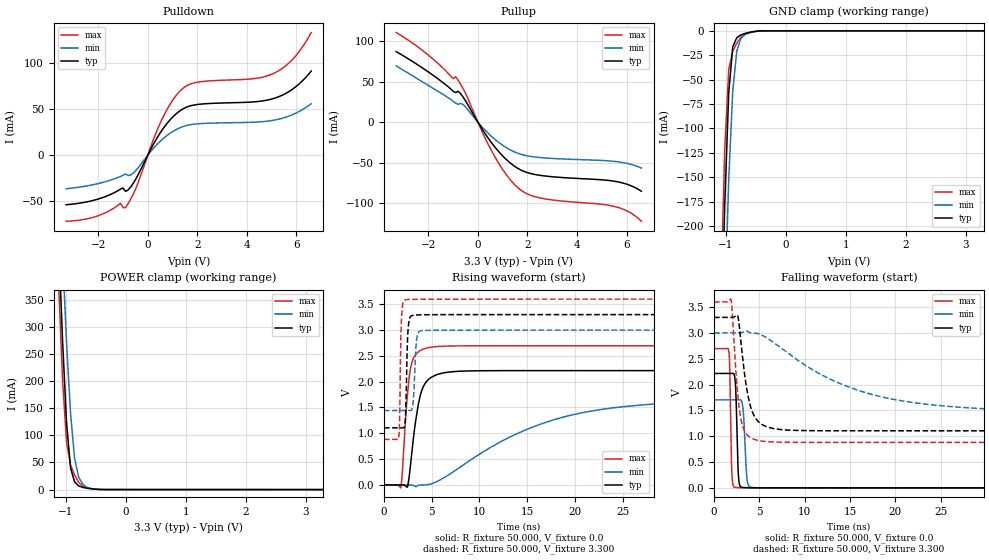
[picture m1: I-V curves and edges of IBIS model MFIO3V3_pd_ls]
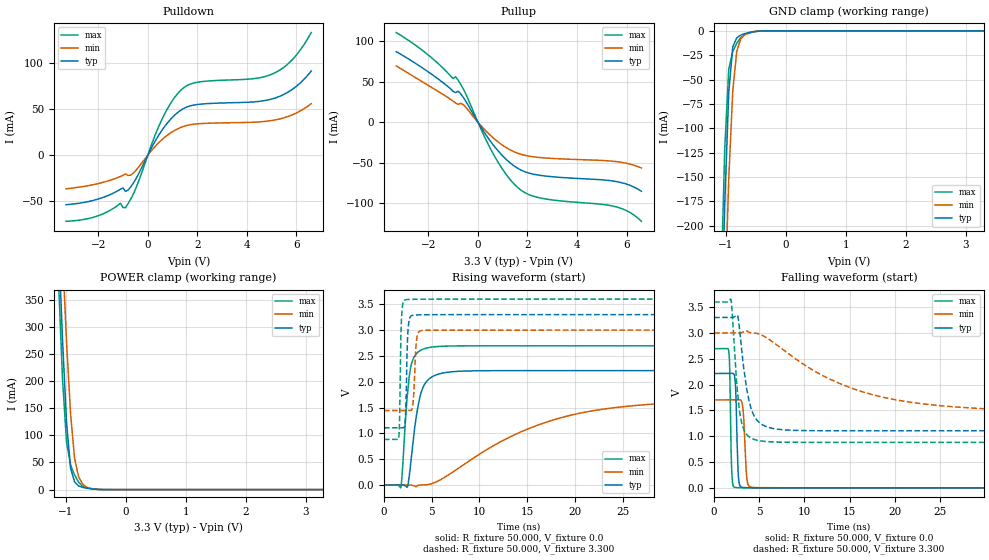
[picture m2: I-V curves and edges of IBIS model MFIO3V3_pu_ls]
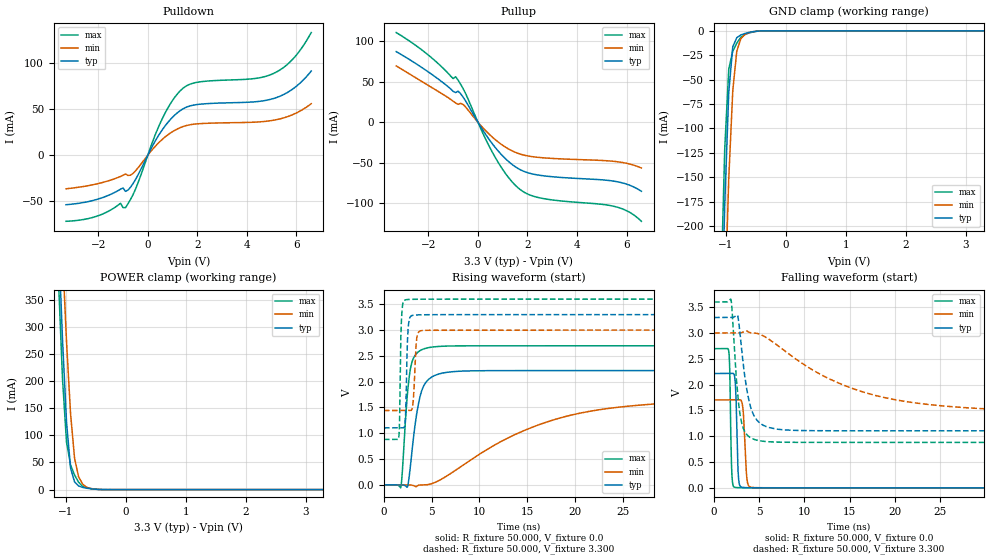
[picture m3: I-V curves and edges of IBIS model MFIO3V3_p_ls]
| IBIS file lpc551x_htqfp64.ibs
[IBIS Ver]   5.0
[File name]   lpc551x_htqfp64.ibs
[File Rev]   1.0
[Date]   June 22,2020
[Notes]   Rev History
|   1.0  initial release
[Disclaimer]   The model given below represents a 64-pin package.
[Copyright]   Copyright NXP 2020
[Component] lpc551x
[Manufacturer] NXP
[Package]
|   typ   min   max
R_pkg   0.19702   0.096175   0.23367
L_pkg   3.574e-9   2.964e-9   4.311e-9
C_pkg   4.829e-13   4.303e-13   6.109e-13
[Pin]   signal_name   model_name   R_pin   L_pin   C_pin
9   VDDA   POWER   NA   NA   NA
25   VBUS   POWER   0.20915   3.347e-9   4.679e-13
27   USB1_3V3   POWER   NA   NA   NA
61   USB0_3V3   POWER   NA   NA   NA
8   VDDE   POWER   NA   NA   NA
16   VDDE   POWER   NA   NA   NA
43   VDDE   POWER   NA   NA   NA
54   VDDE   POWER   NA   NA   NA
28   VDD_PMU   POWER   NA   NA   NA
10   VREFP   POWER   0.18173   2.964e-9   4.54e-13
32   VBAT_DCDC_CORE   POWER   0.096175   3.194e-9   6.109e-13
33   VBAT_PMU   POWER   0.21402   4.013e-9   4.752e-13
24   USB1_DM   NC   0.20325   3.453e-9   4.718e-13
23   USB1_DP   NC   0.21049   3.339e-9   4.746e-13
29   FB   NC   NA   NA   NA
31   LX   NC   0.12749   3.011e-9   5.849e-13
36   P0_0   gpio3v3   0.18524   3.505e-9 4.679e-13
2   P0_1   gpio3v3   0.21276   3.977e-9 5.283e-13
52   P0_2   gpio3v3   0.20828   3.749e-9 4.838e-13
53   P0_3   gpio3v3   0.20955   3.477e-9 4.766e-13
55   P0_4   gpio3v3   0.20447   3.499e-9 4.566e-13
56   P0_5   gpio3v3   0.20052   3.543e-9  4.69e-13
57   P0_6   gpio3v3   0.20007   3.565e-9 4.736e-13
1   P0_7   gpio3v3   0.22847   4.288e-9 5.092e-13
17   P0_8   gpio3v3   0.22136   4.132e-9 4.883e-13
37   P0_9   gpio3v3   0.1773   3.36e-9 4.575e-13
13   P0_10   gpio3v3   0.18906   3.545e-9 4.881e-13
6   P0_11   gpio3v3   0.17925   3.357e-9  4.61e-13
5   P0_12   gpio3v3   0.18582   3.52e-9  4.76e-13
46   P0_13   iicgpio3v3   0.19221   3.582e-9 4.844e-13
47   P0_14   iicgpio3v3   0.20296   3.765e-9 4.948e-13
14   P0_15   gpio3v3   0.19983   3.666e-9 5.083e-13
7   P0_16   gpio3v3   0.17909   3.101e-9 4.519e-13
3   P0_17   gpio3v3   0.20017   3.778e-9 4.971e-13
38   P0_18   gpio3v3   0.17183   3.265e-9 4.388e-13
58   P0_19   gpio3v3   0.20259   3.636e-9 4.686e-13
48   P0_20   gpio3v3   0.21365   4.055e-9 4.764e-13
49   P0_21   gpio3v3   0.22994   4.311e-9 4.976e-13
50   P0_22   gpio3v3   0.2203   4.016e-9 5.173e-13
12   P0_23   gpio3v3   0.1835   3.254e-9 4.662e-13
45   P0_24   gpio3v3   0.18339   3.43e-9 4.615e-13
51   P0_25   gpio3v3   0.21235   3.87e-9 5.028e-13
40   P0_26   gpio3v3   0.16841   3.135e-9 4.403e-13
18   P0_27   gpio3v3   0.21181   3.898e-9 4.964e-13
44   P0_28   gpio3v3   0.18479   3.216e-9 4.418e-13
59   P0_29   gpio3v3   0.20617   3.657e-9  4.73e-13
60   P0_30   gpio3v3   0.21575   3.597e-9 4.783e-13
15   P0_31   gpio3v3   0.21765   3.65e-9 5.199e-13
4   P1_0   gpio3v3   0.19509   3.68e-9 4.803e-13
39   P1_1   gpio3v3   0.16986   3.202e-9 4.303e-13
41   P1_2   gpio3v3   0.17055   3.135e-9 4.429e-13
42   P1_3   gpio3v3   0.17903   3.13e-9 4.331e-13
21   RESETN   gpio3v3   0.21486   3.524e-9 4.684e-13
63   USB0_DM   NC   0.23367   3.701e-9   5.248e-13
62   USB0_DP   NC   0.23063   3.603e-9   5.115e-13
35   XTAL32K_N   NC   0.19233   3.61e-9   4.888e-13
34   XTAL32K_P   NC   0.20386   3.799e-9   5.036e-13
19   XTAL32M_N   NC   0.21308   3.871e-9   4.912e-13
20   XTAL32M_P   NC   0.2074   3.75e-9   4.799e-13
65   VSS   GND   NA   NA   NA
11   VSSA   GND   NA   NA   NA
22   USB1_VSS   GND   NA   NA   NA
26   USB1_VSS   GND   NA   NA   NA
30   VSS_DCDC   GND   NA   NA   NA
64   USB0_VSS   GND   NA   NA   NA
|   Model Selector
[Model Selector] gpio3v3
MFIO3V3_pd_hs  EPUN=1 EPD=1 EHS=1
MFIO3V3_pd_ls  EPUN=1 EPD=1 EHS=0
MFIO3V3_pu_hs  EPUN=0 EPD=0 EHS=1
MFIO3V3_pu_ls  EPUN=0 EPD=0 EHS=0
MFIO3V3_p_hs  EPUN=1 EPD=0 EHS=1
MFIO3V3_p_ls  EPUN=1 EPD=0 EHS=0
MFIO3V3_r_hs  EPUN=0 EPD=1 EHS=1
MFIO3V3_r_ls  EPUN=0 EPD=1 EHS=0
[Model Selector] iicgpio3v3
IIC3V3_pd_hs  EGP=1 EPUN=1 EPD=1 EHS=1
IIC3V3_pd_ls  EGP=1 EPUN=1 EPD=1 EHS=0
IIC3V3_p_hs  EGP=1 EPUN=1 EPD=0 EHS=1
IIC3V3_p_ls  EGP=1 EPUN=1 EPD=0 EHS=0
IIC3V3_pu_hs  EGP=1 EPUN=0 EPD=0 EHS=1
IIC3V3_pu_ls  EGP=1 EPUN=0 EPD=0 EHS=0
IIC3V3_r_hs  EGP=1 EPUN=0 EPD=1 EHS=1
IIC3V3_r_ls  EGP=1 EPUN=0 EPD=1 EHS=0
IIC3V3_pd_iic_hs  EGP=0 ECS=0 EPUN=1 EPD=1
IIC3V3_p_iic_hs  EGP=0 ECS=0 EPUN=1 EPD=0
IIC3V3_pu_iic_hs  EGP=0 ECS=0 EPUN=0 EPD=0
IIC3V3_r_iic_hs  EGP=0 ECS=0 EPUN=0 EPD=1
IIC3V3_pd_iic_pu_hs  EGP=0 ECS=1 EPUN=1 EPD=1  SSEL=1
IIC3V3_p_iic_pu_hs  EGP=0 ECS=1 EPUN=1 EPD=0  SSEL=1
IIC3V3_pu_iic_pu_hs  EGP=0 ECS=1 EPUN=0 EPD=0  SSEL=1
IIC3V3_r_iic_pu_hs  EGP=0 ECS=1 EPUN=0 EPD=1  SSEL=1
| Models and submodels in the file (24): MFIO3V3_pd_hs (I/O), MFIO3V3_pd_ls (I/O), MFIO3V3_pu_hs (I/O), MFIO3V3_pu_ls (I/O), MFIO3V3_p_hs (I/O), MFIO3V3_p_ls (I/O), MFIO3V3_r_hs (I/O), MFIO3V3_r_ls (I/O), IIC3V3_pd_hs (I/O), IIC3V3_pd_ls (I/O), IIC3V3_p_hs (I/O), IIC3V3_p_ls (I/O), IIC3V3_pu_hs (I/O), IIC3V3_pu_ls (I/O), IIC3V3_r_hs (I/O), IIC3V3_r_ls (I/O), IIC3V3_pd_iic_hs (I/O_open_drain), IIC3V3_p_iic_hs (I/O_open_drain), IIC3V3_pu_iic_hs (I/O_open_drain), IIC3V3_r_iic_hs (I/O_open_drain), IIC3V3_pd_iic_pu_hs (I/O_open_drain), IIC3V3_p_iic_pu_hs (I/O_open_drain), IIC3V3_pu_iic_pu_hs (I/O_open_drain), IIC3V3_r_iic_pu_hs (I/O_open_drain)
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|   Model MFIO3V3_pd_ls
[Model] MFIO3V3_pd_ls
Model_type I/O
Polarity   Non-Inverting
Enable   Active-Low
Vinl =  0.990V
Vinh =  2.310V
Vmeas =  1.650V
Cref =  0.0F
Rref =  100.000
Vref =  0.0V
C_comp   1.906pF   1.877pF   1.925pF
C_comp_pullup   1.141pF   1.113pF   1.145pF
C_comp_pulldown   0.641pF   0.601pF   0.647pF
[Model Spec]
Vinh   2.310V   2.100V   2.520V
Vinl   0.990V   0.900V   1.080V
Vmeas   1.650V   1.500V   1.800V
Vref   0.0V   0.0V   0.0V
Cref   0.0F   0.0F   0.0F
Rref   100.000   100.000   100.000
[Temperature Range]   25.000   0.125k   -40.000
[Voltage Range]   3.300V   3.000V   3.600V
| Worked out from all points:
|   slope of the pulldown table from 0 to 0.495 V, typ, clamps not added: 20.7 ohm
|   slope of the pullup table from 0 to 0.495 V, typ, clamps not added: 21.4 ohm
|   GND clamp passes 1 mA (typ) near -0.56 V on its own axis
|   POWER clamp passes 1 mA (typ) near -0.53 V on its own axis
|   rising waveform, R_fixture 50.000, V_fixture 0.0: 20-80 % time 1.05ns typ, 11.9ns min, 670ps max; typ from 0 V to 2.21 V
|   rising waveform, R_fixture 50.000, V_fixture 3.300: 20-80 % time 176ps typ, 234ps min, 146ps max; typ from 1.1 V to 3.3 V
|   falling waveform, R_fixture 50.000, V_fixture 0.0: 20-80 % time 203ps typ, 279ps min, 162ps max; typ from 2.21 V to 0 V
|   falling waveform, R_fixture 50.000, V_fixture 3.300: 20-80 % time 1.13ns typ, 11.2ns min, 744ps max; typ from 3.3 V to 1.1 V
[Pulldown]
|Voltage   I(typ)   I(min)   I(max)
-3.3V     -53.7mA    -36.43mA   -71.67mA
-2.1V     -48.29mA   -31.37mA   -66.51mA
-1.1V     -36.82mA   -23.05mA   -52.1mA
-900mV    -39.2mA    -20.39mA   -56.91mA
-600mV    -30.96mA   -19.83mA   -42.97mA
600mV     28.07mA    17.5mA     40.4mA
1V        41.17mA    25.53mA    59.41mA
1.4V      49.87mA    30.79mA    72.04mA
2V        54.93mA    33.94mA    79.03mA
5V        60.84mA    37.53mA    87.68mA
5.9V      72.62mA    44.52mA    105.4mA
6.6V      91.19mA    55.78mA    132.9mA
[Pullup]
|Voltage   I(typ)   I(min)   I(max)
-3.3V     87.16mA    69.54mA    110.7mA
-2.1V     64.12mA    47.22mA    85.31mA
-1V       38.1mA     25.85mA    53.88mA
-900mV    36.64mA    23.75mA    56.16mA
-800mV    38.25mA    22.02mA    51.93mA
-600mV    31.06mA    21.93mA    41.58mA
700mV     -31.25mA   -21.55mA   -43.56mA
1.2V      -47.6mA    -32.42mA   -66.97mA
1.7V      -58.52mA   -39.3mA    -83.05mA
2.6V      -66.01mA   -43.88mA   -94.06mA
5.6V      -73.4mA    -48.74mA   -104.7mA
6.6V      -85.32mA   -56.6mA    -122.4mA
[GND_clamp]
|Voltage   I(typ)   I(min)   I(max)
-3.3V     -7.222A    -7.177A    -7.278A
-1.089V   -337.1mA   -440.8mA   -274.1mA
-1.022V   -178.2mA   -284.2mA   -121mA
-955mV    -63.05mA   -151.6mA   -39.25mA
-888mV    -16.33mA   -61.34mA   -20.9mA
-821mV    -7.066mA   -20.84mA   -12.66mA
-754mV    -4.265mA   -8.157mA   -6.693mA
-687mV    -2.794mA   -3.896mA   -3.841mA
-620mV    -1.725mA   -1.894mA   -2.339mA
-419mV    -112.4uA   -138.2uA   -135uA
3.3V      0A         0A         0A
[POWER_clamp]
|Voltage   I(typ)   I(min)   I(max)
-3.3V     8.016A     7.986A     8.074A
-1.122V   463.8mA    614.4mA    385mA
-1.055V   276.3mA    435mA      203.9mA
-988mV    124.1mA    272.4mA    87.22mA
-921mV    40.03mA    140.2mA    45.68mA
-854mV    14.24mA    57.83mA    27.12mA
-787mV    6.921mA    23.8mA     13.77mA
-720mV    4.141mA    10.27mA    6.207mA
-653mV    2.682mA    4.42mA     3.699mA
-586mV    1.616mA    1.919mA    2.191mA
-452mV    346.9uA    411.9uA    422.9uA
3.3V      0A         0A         0A
[Ramp]
| variable   typ   min   max
dV/dt_r   1.328/1.048n   1.021/11.887n   1.617/0.670n
dV/dt_f   1.317/1.132n   0.935/11.171n   1.631/0.743n
R_load = 50.000
[Rising Waveform]
R_fixture= 50.000
V_fixture= 0.0
V_fixture_min= 0.0
V_fixture_max= 0.0
|time   V(typ)   V(min)   V(max)
0s        11.38nV    124.8nV    46.5nV
1.76ns    11.77uV    -379.4nV   -52.39mV
1.89ns    124.5uV    -254.1nV   156mV
2.47ns    -34.09mV   65.71uV    1.767V
2.93ns    642.6mV    -4.824mV   2.378V
3.75ns    1.693V     -3.224mV   2.598V
4.9ns     2.078V     17.79mV    2.667V
15.38ns   2.214V     1.106V     2.695V
25.84ns   2.214V     1.529V     2.695V
100ns     2.214V     1.702V     2.695V
[Rising Waveform]
R_fixture= 50.000
V_fixture= 3.300
V_fixture_min= 3.000
V_fixture_max= 3.600
|time   V(typ)   V(min)   V(max)
0s        1.105V     1.44V      880.4mV
1.55ns    1.105V     1.44V      919.2mV
1.85ns    1.105V     1.44V      3.271V
2.2ns     1.184V     1.44V      3.582V
2.34ns    1.855V     1.44V      3.589V
2.64ns    3.192V     1.44V      3.594V
3.07ns    3.287V     1.621V     3.596V
3.43ns    3.293V     2.839V     3.597V
4.06ns    3.296V     2.992V     3.598V
100ns     3.299V     2.999V     3.599V
[Falling Waveform]
R_fixture= 50.000
V_fixture= 0.0
V_fixture_min= 0.0
V_fixture_max= 0.0
|time   V(typ)   V(min)   V(max)
0s        2.214V     1.703V     2.695V
1.63ns    2.214V     1.703V     2.64V
1.73ns    2.214V     1.703V     2.3V
1.97ns    2.214V     1.703V     263mV
2.38ns    1.941V     1.702V     7.184mV
2.7ns     199.7mV    1.703V     3.012mV
3.2ns     7.193mV    1.527V     1.541mV
3.63ns    2.938mV    178.8mV    1.008mV
4.26ns    1.462mV    6.421mV    552.8uV
100ns     15.88nV    209.7nV    49.27nV
[Falling Waveform]
R_fixture= 50.000
V_fixture= 3.300
V_fixture_min= 3.000
V_fixture_max= 3.600
|time   V(typ)   V(min)   V(max)
0s        3.299V     2.999V     3.599V
1.87ns    3.299V     2.999V     3.646V
2.6ns     3.336V     2.999V     1.836V
3.1ns     2.603V     3.009V     1.222V
3.85ns    1.693V     3.011V     992.4mV
4.41ns    1.398V     2.998V     939.4mV
5.16ns    1.242V     2.965V     908.2mV
14.39ns   1.105V     1.984V     880.4mV
25.09ns   1.105V     1.589V     880.4mV
100ns     1.105V     1.44V      880.4mV
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|   Model MFIO3V3_pu_ls
[Model] MFIO3V3_pu_ls
Model_type I/O
Polarity   Non-Inverting
Enable   Active-Low
Vinl =  0.990V
Vinh =  2.310V
Vmeas =  1.650V
Cref =  0.0F
Rref =  100.000
Vref =  0.0V
C_comp   1.906pF   1.877pF   1.925pF
C_comp_pullup   1.139pF   1.112pF   1.144pF
C_comp_pulldown   0.643pF   0.602pF   0.649pF
[Model Spec]
Vinh   2.310V   2.100V   2.520V
Vinl   0.990V   0.900V   1.080V
Vmeas   1.650V   1.500V   1.800V
Vref   0.0V   0.0V   0.0V
Cref   0.0F   0.0F   0.0F
Rref   100.000   100.000   100.000
[Temperature Range]   25.000   0.125k   -40.000
[Voltage Range]   3.300V   3.000V   3.600V
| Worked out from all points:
|   slope of the pulldown table from 0 to 0.495 V, typ, clamps not added: 20.7 ohm
|   slope of the pullup table from 0 to 0.495 V, typ, clamps not added: 21.4 ohm
|   GND clamp passes 1 mA (typ) near -0.55 V on its own axis
|   POWER clamp passes 1 mA (typ) near -0.54 V on its own axis
|   rising waveform, R_fixture 50.000, V_fixture 0.0: 20-80 % time 1.05ns typ, 11.9ns min, 674ps max; typ from 0.001 V to 2.21 V
|   rising waveform, R_fixture 50.000, V_fixture 3.300: 20-80 % time 179ps typ, 230ps min, 146ps max; typ from 1.11 V to 3.3 V
|   falling waveform, R_fixture 50.000, V_fixture 0.0: 20-80 % time 203ps typ, 278ps min, 162ps max; typ from 2.21 V to 0.001 V
|   falling waveform, R_fixture 50.000, V_fixture 3.300: 20-80 % time 1.14ns typ, 11.2ns min, 744ps max; typ from 3.3 V to 1.11 V
[Pulldown]
|Voltage   I(typ)   I(min)   I(max)
-3.3V     -53.7mA    -36.43mA   -71.67mA
-2.1V     -48.29mA   -31.37mA   -66.51mA
-1.1V     -36.82mA   -23.05mA   -52.1mA
-900mV    -39.2mA    -20.39mA   -56.91mA
-600mV    -30.96mA   -19.83mA   -42.97mA
600mV     28.07mA    17.5mA     40.4mA
1V        41.17mA    25.53mA    59.41mA
1.4V      49.87mA    30.79mA    72.04mA
2V        54.93mA    33.94mA    79.03mA
5V        60.84mA    37.53mA    87.68mA
5.9V      72.62mA    44.52mA    105.4mA
6.6V      91.19mA    55.78mA    132.9mA
[Pullup]
|Voltage   I(typ)   I(min)   I(max)
-3.3V     87.16mA    69.54mA    110.7mA
-2.1V     64.12mA    47.22mA    85.31mA
-1V       38.1mA     25.85mA    53.88mA
-900mV    36.64mA    23.75mA    56.16mA
-800mV    38.25mA    22.02mA    51.93mA
-600mV    31.06mA    21.93mA    41.58mA
700mV     -31.25mA   -21.55mA   -43.56mA
1.2V      -47.6mA    -32.42mA   -66.97mA
1.7V      -58.52mA   -39.3mA    -83.05mA
2.6V      -66.01mA   -43.88mA   -94.06mA
5.6V      -73.4mA    -48.74mA   -104.7mA
6.6V      -85.32mA   -56.6mA    -122.4mA
[GND_clamp]
|Voltage   I(typ)   I(min)   I(max)
-3.3V     -7.222A    -7.177A    -7.278A
-1.089V   -337.2mA   -440.9mA   -274.2mA
-1.022V   -178.3mA   -284.2mA   -121.1mA
-955mV    -63.12mA   -151.7mA   -39.33mA
-888mV    -16.39mA   -61.39mA   -20.98mA
-821mV    -7.132mA   -20.89mA   -12.74mA
-754mV    -4.331mA   -8.209mA   -6.777mA
-687mV    -2.86mA    -3.948mA   -3.925mA
-620mV    -1.791mA   -1.946mA   -2.423mA
-419mV    -178.1uA   -190.3uA   -219.1uA
3.3V      0A         0A         0A
[POWER_clamp]
|Voltage   I(typ)   I(min)   I(max)
-3.3V     8.016A     7.986A     8.074A
-1.122V   463.7mA    614.3mA    385mA
-1.055V   276.3mA    434.9mA    203.9mA
-988mV    124mA      272.3mA    87.13mA
-921mV    39.96mA    140.1mA    45.6mA
-854mV    14.17mA    57.77mA    27.03mA
-787mV    6.855mA    23.75mA    13.68mA
-720mV    4.075mA    10.22mA    6.123mA
-653mV    2.616mA    4.368mA    3.615mA
-586mV    1.55mA     1.867mA    2.107mA
-452mV    281.1uA    359.9uA    338.7uA
3.3V      0A         0A         0A
[Ramp]
| variable   typ   min   max
dV/dt_r   1.329/1.048n   1.022/11.881n   1.617/0.670n
dV/dt_f   1.316/1.133n   0.935/11.179n   1.631/0.744n
R_load = 50.000
[Rising Waveform]
R_fixture= 50.000
V_fixture= 0.0
V_fixture_min= 0.0
V_fixture_max= 0.0
|time   V(typ)   V(min)   V(max)
0s        869.8uV    949.2uV    842.8uV
1.76ns    883.1uV    948.8uV    -50.04mV
1.91ns    1.009mV    949.1uV    208mV
2.46ns    -36.02mV   1.012mV    1.752V
2.89ns    574.4mV    -2.122mV   2.352V
3.71ns    1.664V     -1.354mV   2.595V
4.93ns    2.083V     22.11mV    2.669V
15.41ns   2.215V     1.111V     2.696V
25.89ns   2.215V     1.532V     2.696V
100ns     2.215V     1.704V     2.696V
[Rising Waveform]
R_fixture= 50.000
V_fixture= 3.300
V_fixture_min= 3.000
V_fixture_max= 3.600
|time   V(typ)   V(min)   V(max)
0s        1.106V     1.442V     881.7mV
1.55ns    1.106V     1.442V     920.7mV
1.83ns    1.106V     1.442V     3.201V
2.2ns     1.19V      1.442V     3.584V
2.36ns    2.014V     1.442V     3.591V
2.67ns    3.219V     1.441V     3.595V
3.05ns    3.288V     1.591V     3.597V
3.47ns    3.295V     2.885V     3.598V
4.05ns    3.297V     2.994V     3.599V
100ns     3.3V       3V         3.6V
[Falling Waveform]
R_fixture= 50.000
V_fixture= 0.0
V_fixture_min= 0.0
V_fixture_max= 0.0
|time   V(typ)   V(min)   V(max)
0s        2.215V     1.704V     2.696V
1.63ns    2.215V     1.704V     2.641V
1.73ns    2.215V     1.704V     2.3V
1.97ns    2.216V     1.704V     265.9mV
2.37ns    1.988V     1.704V     8.752mV
2.68ns    252.6mV    1.704V     4.211mV
3.22ns    8.138mV    1.493V     2.448mV
3.64ns    3.966mV    165.1mV    1.883mV
4.28ns    2.4mV      8.68mV     1.408mV
100ns     869.8uV    949.4uV    842.8uV
[Falling Waveform]
R_fixture= 50.000
V_fixture= 3.300
V_fixture_min= 3.000
V_fixture_max= 3.600
|time   V(typ)   V(min)   V(max)
0s        3.3V       3V         3.6V
1.88ns    3.3V       3V         3.639V
2.61ns    3.334V     3V         1.817V
3.06ns    2.664V     3.008V     1.251V
3.83ns    1.711V     3.015V     996.5mV
4.37ns    1.414V     3.001V     943.5mV
5.06ns    1.258V     2.975V     912.3mV
14.38ns   1.106V     1.987V     881.7mV
25.08ns   1.106V     1.591V     881.7mV
100ns     1.106V     1.442V     881.7mV
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|   Model MFIO3V3_p_ls
[Model] MFIO3V3_p_ls
Model_type I/O
Polarity   Non-Inverting
Enable   Active-Low
Vinl =  0.990V
Vinh =  2.310V
Vmeas =  1.650V
Cref =  0.0F
Rref =  100.000
Vref =  0.0V
C_comp   1.906pF   1.877pF   1.925pF
C_comp_pullup   1.140pF   1.112pF   1.144pF
C_comp_pulldown   0.642pF   0.602pF   0.649pF
[Model Spec]
Vinh   2.310V   2.100V   2.520V
Vinl   0.990V   0.900V   1.080V
Vmeas   1.650V   1.500V   1.800V
Vref   0.0V   0.0V   0.0V
Cref   0.0F   0.0F   0.0F
Rref   100.000   100.000   100.000
[Temperature Range]   25.000   0.125k   -40.000
[Voltage Range]   3.300V   3.000V   3.600V
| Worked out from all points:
|   slope of the pulldown table from 0 to 0.495 V, typ, clamps not added: 20.7 ohm
|   slope of the pullup table from 0 to 0.495 V, typ, clamps not added: 21.4 ohm
|   GND clamp passes 1 mA (typ) near -0.56 V on its own axis
|   POWER clamp passes 1 mA (typ) near -0.54 V on its own axis
|   rising waveform, R_fixture 50.000, V_fixture 0.0: 20-80 % time 1.05ns typ, 11.9ns min, 670ps max; typ from 0 V to 2.21 V
|   rising waveform, R_fixture 50.000, V_fixture 3.300: 20-80 % time 177ps typ, 237ps min, 147ps max; typ from 1.1 V to 3.3 V
|   falling waveform, R_fixture 50.000, V_fixture 0.0: 20-80 % time 203ps typ, 282ps min, 162ps max; typ from 2.21 V to 0 V
|   falling waveform, R_fixture 50.000, V_fixture 3.300: 20-80 % time 1.14ns typ, 11.2ns min, 740ps max; typ from 3.3 V to 1.1 V
[Pulldown]
|Voltage   I(typ)   I(min)   I(max)
-3.3V     -53.7mA    -36.43mA   -71.67mA
-2.1V     -48.29mA   -31.37mA   -66.51mA
-1.1V     -36.82mA   -23.05mA   -52.1mA
-900mV    -39.2mA    -20.39mA   -56.91mA
-600mV    -30.96mA   -19.83mA   -42.97mA
600mV     28.07mA    17.5mA     40.4mA
1V        41.17mA    25.53mA    59.41mA
1.4V      49.87mA    30.79mA    72.04mA
2V        54.93mA    33.94mA    79.03mA
5V        60.84mA    37.53mA    87.68mA
5.9V      72.62mA    44.52mA    105.4mA
6.6V      91.19mA    55.78mA    132.9mA
[Pullup]
|Voltage   I(typ)   I(min)   I(max)
-3.3V     87.16mA    69.54mA    110.7mA
-2.1V     64.12mA    47.22mA    85.31mA
-1V       38.1mA     25.85mA    53.88mA
-900mV    36.64mA    23.75mA    56.16mA
-800mV    38.25mA    22.02mA    51.93mA
-600mV    31.06mA    21.93mA    41.58mA
700mV     -31.25mA   -21.55mA   -43.56mA
1.2V      -47.6mA    -32.42mA   -66.97mA
1.7V      -58.52mA   -39.3mA    -83.05mA
2.6V      -66.01mA   -43.88mA   -94.06mA
5.6V      -73.4mA    -48.74mA   -104.7mA
6.6V      -85.32mA   -56.6mA    -122.4mA
[GND_clamp]
|Voltage   I(typ)   I(min)   I(max)
-3.3V     -7.222A    -7.177A    -7.278A
-1.089V   -337.1mA   -440.8mA   -274.1mA
-1.022V   -178.2mA   -284.2mA   -121mA
-955mV    -63.04mA   -151.6mA   -39.24mA
-888mV    -16.32mA   -61.33mA   -20.89mA
-821mV    -7.057mA   -20.83mA   -12.64mA
-754mV    -4.256mA   -8.15mA    -6.682mA
-687mV    -2.785mA   -3.888mA   -3.83mA
-620mV    -1.717mA   -1.887mA   -2.329mA
-419mV    -104.8uA   -131.8uA   -126uA
3.3V      0A         0A         0A
[POWER_clamp]
|Voltage   I(typ)   I(min)   I(max)
-3.3V     8.016A     7.986A     8.074A
-1.122V   463.7mA    614.3mA    384.9mA
-1.055V   276.2mA    434.9mA    203.8mA
-988mV    124mA      272.3mA    87.12mA
-921mV    39.95mA    140.1mA    45.59mA
-854mV    14.16mA    57.77mA    27.02mA
-787mV    6.846mA    23.74mA    13.67mA
-720mV    4.066mA    10.21mA    6.113mA
-653mV    2.607mA    4.361mA    3.605mA
-586mV    1.542mA    1.86mA     2.097mA
-452mV    273.4uA    353.7uA    329.6uA
3.3V      0A         0A         0A
[Ramp]
| variable   typ   min   max
dV/dt_r   1.329/1.049n   1.022/11.884n   1.618/0.670n
dV/dt_f   1.317/1.134n   0.935/11.178n   1.632/0.744n
R_load = 50.000
[Rising Waveform]
R_fixture= 50.000
V_fixture= 0.0
V_fixture_min= 0.0
V_fixture_max= 0.0
|time   V(typ)   V(min)   V(max)
0s        11.91nV    127.2nV    48.18nV
1.76ns    14.07uV    -353.2nV   -52.48mV
1.9ns     130.3uV    -106.1nV   185.6mV
2.46ns    -38.99mV   62.57uV    1.761V
2.93ns    644.9mV    -4.797mV   2.378V
3.65ns    1.606V     -5.408mV   2.586V
4.94ns    2.084V     20.24mV    2.669V
15.63ns   2.215V     1.125V     2.696V
25.83ns   2.215V     1.53V      2.696V
100ns     2.215V     1.703V     2.696V
[Rising Waveform]
R_fixture= 50.000
V_fixture= 3.300
V_fixture_min= 3.000
V_fixture_max= 3.600
|time   V(typ)   V(min)   V(max)
0s        1.105V     1.441V     880.7mV
1.55ns    1.105V     1.441V     919.6mV
1.84ns    1.105V     1.441V     3.233V
2.22ns    1.224V     1.441V     3.584V
2.37ns    2.139V     1.441V     3.59V
2.68ns    3.224V     1.44V      3.594V
3.06ns    3.287V     1.603V     3.596V
3.45ns    3.294V     2.861V     3.598V
4.07ns    3.297V     2.993V     3.599V
100ns     3.3V       3V         3.6V
[Falling Waveform]
R_fixture= 50.000
V_fixture= 0.0
V_fixture_min= 0.0
V_fixture_max= 0.0
|time   V(typ)   V(min)   V(max)
0s        2.215V     1.703V     2.696V
1.62ns    2.215V     1.703V     2.651V
1.73ns    2.215V     1.703V     2.303V
1.97ns    2.215V     1.703V     265.7mV
2.37ns    1.981V     1.703V     8.251mV
2.69ns    225.2mV    1.704V     3.621mV
3.22ns    7.595mV    1.492V     1.863mV
3.64ns    3.369mV    166.1mV    1.261mV
4.27ns    1.779mV    7.484mV    732uV
100ns     16.41nV    212.2nV    50.94nV
[Falling Waveform]
R_fixture= 50.000
V_fixture= 3.300
V_fixture_min= 3.000
V_fixture_max= 3.600
|time   V(typ)   V(min)   V(max)
0s        3.3V       3V         3.6V
1.88ns    3.3V       3V         3.641V
2.61ns    3.334V     3V         1.821V
3.08ns    2.642V     3.009V     1.24V
3.83ns    1.711V     3.015V     995.8mV
4.38ns    1.41V      3.001V     942.3mV
5.17ns    1.242V     2.968V     908.5mV
14.42ns   1.105V     1.984V     880.8mV
25.12ns   1.105V     1.59V      880.7mV
100ns     1.105V     1.441V     880.7mV
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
